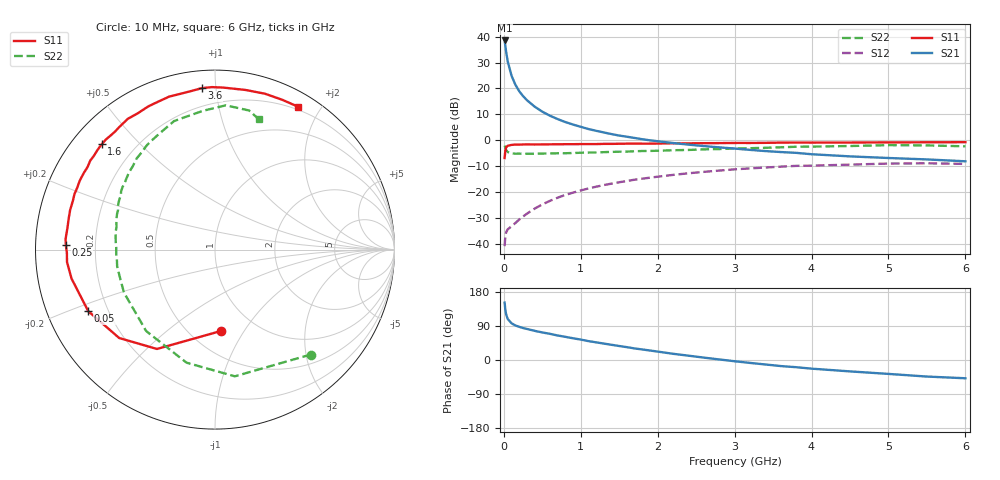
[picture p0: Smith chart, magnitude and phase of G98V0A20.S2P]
! SIEMENS Small Signal Semiconductors
! BFG235
! Si NPN RF Bipolar Junction Transistor in SOT223
! VCE = 8 V  IC = 200 mA
! Common Emitter S-Parameters:  July  1994
# GHz  S  MA  R  50
!  f  S11  S21  S12  S22
! GHz  MAG  ANG  MAG  ANG  MAG  ANG  MAG  ANG
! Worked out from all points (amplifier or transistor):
!   40 points, 10 MHz to 6 GHz, reference 50 ohm
!   highest |S21| = 38.5 dB at 10 MHz (marker M1)
!   |S21| within 3 dB of that: start of sweep to 23.67 MHz
!   unconditionally stable (mu >= 1): 442.8 MHz to 1.509 GHz
!   at 200 MHz: K = 0.82, MSG = 24.7 dB, |S12| = -30.5 dB
!   at 1.5 GHz: K = 1.00, MAG = 8.8 dB, |S12| = -16.2 dB
!   at 6 GHz: K = 0.89, MSG = 0.5 dB, |S12| = -9.1 dB
!   S11 on the Smith chart (normalised r, x): 10 MHz: 0.69, -0.79; 50 MHz: 0.13, -0.23; 250 MHz: 0.09, +0.01; 1.6 GHz: 0.09, +0.39; 3.6 GHz: 0.09, +0.92; 6 GHz: 0.16, +1.72
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0.01  0.4552 -86.1  84.16 151.3  0.0091 60.5  0.7916 -47.6
0.02  0.6412 -120.3  65.42 132.0  0.0144 47.6  0.7146 -81.1
0.03  0.7264 -137.3  50.71 120.4  0.0168 39.8  0.6496 -104.1
0.05  0.7851 -154.1  33.47 108.3  0.0192 34.1  0.5942 -130.2
0.1  0.8155 -168.6  17.59 96.9  0.022 37.8  0.561 -154.8
0.15  0.8275 -175.2  11.8 91.1  0.0254 44.1  0.5516 -165.0
0.2  0.8254 -178.7  8.832 87.5  0.0297 49.6  0.5531 -170.4
0.25  0.8315 178.3  7.114 84.4  0.0339 53.0  0.5494 -174.1
0.3  0.8345 175.9  5.939 81.9  0.0385 55.8  0.5509 -177.3
0.4  0.8309 171.4  4.464 77.0  0.0481 58.9  0.5506 178.6
0.5  0.8334 167.9  3.567 72.7  0.0581 60.5  0.5551 175.3
0.6  0.8367 164.7  2.976 69.0  0.0681 60.7  0.5587 172.1
0.7  0.8372 161.1  2.565 64.7  0.0784 60.5  0.5621 169.4
0.9  0.8415 155.7  2.012 57.3  0.098 58.4  0.5693 164.8
1.1  0.8466 149.5  1.649 49.8  0.118 55.9  0.5808 160.0
1.6  0.8619 137.1  1.172 33.9  0.1645 47.5  0.6054 149.9
2.2  0.8757 123.7  0.887 16.4  0.2154 36.5  0.6438 138.2
3.2  0.8891 102.6  0.654 -7.7  0.2875 17.2  0.7042 119.6
3.6  0.9026 94.6  0.594 -16.0  0.3104 8.8  0.733 111.4
4.5  0.9056 79.1  0.49 -30.1  0.3396 -7.5  0.7762 94.9
5.5  0.9149 65.8  0.428 -43.7  0.3607 -25.8  0.7979 76.2
6  0.9206 60.0  0.394 -48.2  0.3507 -32.7  0.7655 71.3
